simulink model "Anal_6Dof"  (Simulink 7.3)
settings: Solver=ode45  StartTime=0.0  StopTime=500  RelTol=1e-3
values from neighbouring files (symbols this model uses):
  calfa = cos(alfa0*d2r)    [run.m]
  d2r = pi/180    (= 0.0174532925199)    [run.m]
  Kfilt = (wd1^2*wd2^2*wd3^2*wd4^2*wd5^2*wd6^2)/(wn1^2*wn2^2*wn3^2*wn4^2*wn5^2*wn6^2)    (= 0.818930549142)    [run.m]
  klr = lqr(Ap4,Bp4,Q,R)    [run.m]
  kls = lqr(Ap3,Bp3,Q,R)    [run.m]
  salfa = sin(alfa0*d2r)    [run.m]
  Thet0 = 43    [run.m]
  V0 = 18640    [run.m]
  wd1 = 29    [run.m]
  wd2 = 37    [run.m]
  wd3 = 40    [run.m]
  wd4 = 48    [run.m]
  wd5 = 63    [run.m]
  wd6 = 68    [run.m]
  wd7 = 34    [run.m]
  wd8 = 19.1    [run.m]
  wlp = 6.6    [run.m]
  wlp2 = 12    [run.m]
  wlpr = 12    [run.m]
  wn1 = 30    [run.m]
  wn2 = 37.9    [run.m]
  wn3 = 40.2    [run.m]
  wn4 = 48.6    [run.m]
  wn5 = 64    [run.m]
  wn6 = 68.6    [run.m]
  wn7 = 34    [run.m]
  wn8 = 19.1    [run.m]
  zd1 = 0.12    [run.m]
  zd2 = 0.12    [run.m]
  zd3 = 0.1    [run.m]
  zd4 = 0.1    [run.m]
  zd5 = 0.1    [run.m]
  zd6 = 0.1    [run.m]
  zd7 = 0.1    [run.m]
  zd8 = 0.1    [run.m]
  zlp = 0.9    [run.m]
  zlp2 = 0.7    [run.m]
  zlpr = 0.7    [run.m]
  zn1 = 0.008    [run.m]
  zn2 = 0.01    [run.m]
  zn3 = 0.01    [run.m]
  zn4 = 0.02    [run.m]
  zn5 = 0.01    [run.m]
  zn6 = 0.01    [run.m]
  zn7 = 0.01    [run.m]
  zn8 = 0.01    [run.m]
undefined symbols (not defined in the file or in its folder): Aai, Aao, Af, Bai, Bao, Bf, Cai, Cao, Cf, Dai, Dao, Df, KJmix, KSmix

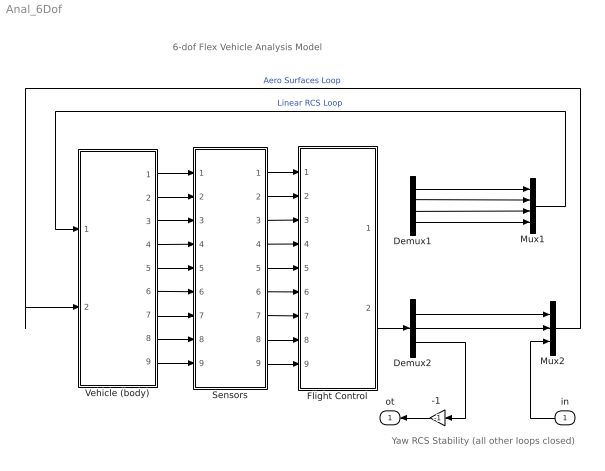
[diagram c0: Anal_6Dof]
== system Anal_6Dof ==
  note: 6-dof Flex Vehicle Analysis Model
  note: Yaw RCS Stability (all other loops closed)
  in : Inport  OutDataType=sfix(16)  OutScaling=2^0
  "-1 " : Gain  Gain=-1  ParameterDataType=sfix(16)  ParameterScaling=2^0  OutDataType=sfix(16)  OutScaling=2^0
  Demux1 : Demux
  Demux2 : Demux  Outputs=3
  Flight Control : Subsystem
  Mux1 : Mux
  Mux2 : Mux  Inputs=3
  Sensors : Subsystem
  Vehicle (body) : Subsystem
  ot : Outport  OutDataType=sfix(16)  OutScaling=2^0
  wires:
  Flight Control/2(Aer_pqr) -> Demux2/1
  Mux2/1 -> Vehicle (body)/2(Aer_pqr)  "Aero Surfaces Loop"
  Mux1/1 -> Vehicle (body)/1(Jet_PQR_Nz)  "Linear RCS Loop"
  Vehicle (body)/1(phi) -> Sensors/1(phi)
  Vehicle (body)/2(p) -> Sensors/2(pb)
  Vehicle (body)/3(r) -> Sensors/3(rb)
  Vehicle (body)/4(bet) -> Sensors/4(beta)
  Vehicle (body)/5(thet) -> Sensors/5(thet)
  Vehicle (body)/6(q) -> Sensors/6(q)
  Vehicle (body)/7(alf) -> Sensors/7(alfa)
  Vehicle (body)/8(Ny) -> Sensors/8(Ny)
  Vehicle (body)/9(Nz) -> Sensors/9(Nz)
  Sensors/1(phio) -> Flight Control/1(phi)
  Sensors/2(pbo) -> Flight Control/2(pb)
  Sensors/3(rbo) -> Flight Control/3(rb)
  Sensors/4(beto) -> Flight Control/4(beta)
  Sensors/5(theto) -> Flight Control/5(thet)
  Sensors/6(qo) -> Flight Control/6(q)
  Sensors/7(alfo) -> Flight Control/7(alfa)
  Sensors/8(Nyo) -> Flight Control/8(Ny)
  Sensors/9(Nzo) -> Flight Control/9(Nz)
  "-1 "/1 -> ot/1
  Demux1/4 -> Mux1/4
  Demux1/1 -> Mux1/1
  Demux2/2 -> Mux2/2
  Demux2/1 -> Mux2/1
  Demux1/2 -> Mux1/2
  Demux2/3 -> "-1 "/1
  in/1 -> Mux2/3
  Demux1/3 -> Mux1/3

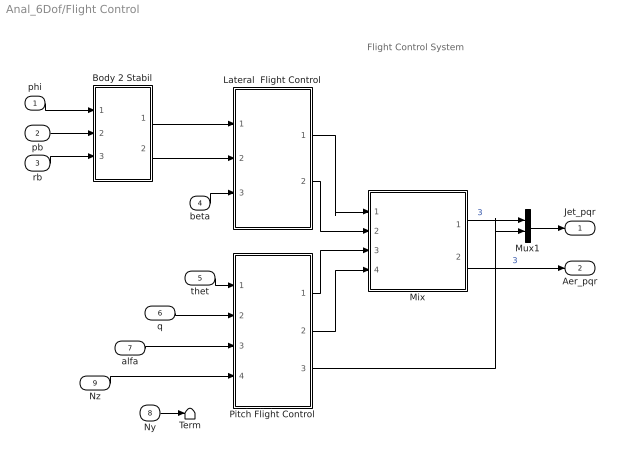
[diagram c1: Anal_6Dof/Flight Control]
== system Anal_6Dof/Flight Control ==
  note: Flight Control System
  phi : Inport  OutDataType=sfix(16)  OutScaling=2^0
  pb : Inport  Port=2  OutDataType=sfix(16)  OutScaling=2^0
  rb : Inport  Port=3  OutDataType=sfix(16)  OutScaling=2^0
  beta : Inport  Port=4  OutDataType=sfix(16)  OutScaling=2^0
  thet : Inport  Port=5  OutDataType=sfix(16)  OutScaling=2^0
  q : Inport  Port=6  OutDataType=sfix(16)  OutScaling=2^0
  alfa : Inport  Port=7  OutDataType=sfix(16)  OutScaling=2^0
  Ny : Inport  Port=8  OutDataType=sfix(16)  OutScaling=2^0
  Nz : Inport  Port=9  OutDataType=sfix(16)  OutScaling=2^0
  Body 2 Stabil : Subsystem
  Lateral  Flight Control : Subsystem
  Mix : Subsystem
  Mux1 : Mux  Inputs=[3,1]
  Pitch Flight Control : Subsystem
  Term : Terminator
  Jet_pqr : Outport  OutDataType=sfix(16)  OutScaling=2^0
  Aer_pqr : Outport  Port=2  OutDataType=sfix(16)  OutScaling=2^0
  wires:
  Lateral  Flight Control/1(rcs_PR) -> Mix/1(Rcs_PR)
  Lateral  Flight Control/2(aero_PR) -> Mix/2(Aer_PR)
  Pitch Flight Control/1(rcs_Q) -> Mix/3(Rcs_Q)
  Pitch Flight Control/2(aero_Q) -> Mix/4(Aer_Q)
  beta/1 -> Lateral  Flight Control/3(beta)
  Mix/2(Aer_pqr) -> Aer_pqr/1  "3"
  thet/1 -> Pitch Flight Control/1(thet)
  q/1 -> Pitch Flight Control/2(q)
  alfa/1 -> Pitch Flight Control/3(alf)
  Body 2 Stabil/2(r_s) -> Lateral  Flight Control/2(rs)
  Body 2 Stabil/1(p_s) -> Lateral  Flight Control/1(ps)
  rb/1 -> Body 2 Stabil/3(r_b)
  pb/1 -> Body 2 Stabil/2(p_b)
  phi/1 -> Body 2 Stabil/1(phi)
  Nz/1 -> Pitch Flight Control/4(Nz)
  Mix/1(Jet_pqr) -> Mux1/1  "3"
  Pitch Flight Control/3(Nzfb) -> Mux1/2
  Mux1/1 -> Jet_pqr/1
  Ny/1 -> Term/1

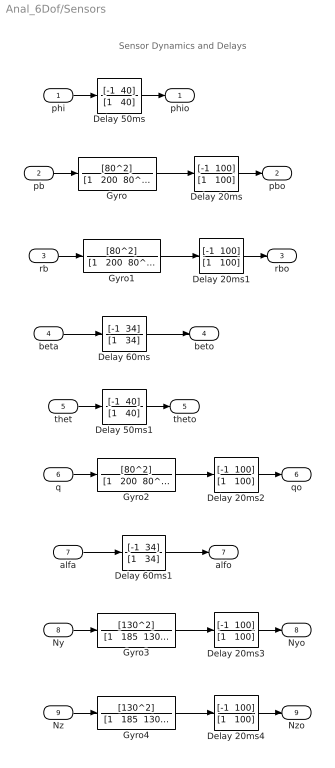
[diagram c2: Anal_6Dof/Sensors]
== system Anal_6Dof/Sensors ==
  note: Sensor Dynamics and Delays
  phi : Inport  OutDataType=sfix(16)  OutScaling=2^0
  pb : Inport  Port=2  OutDataType=sfix(16)  OutScaling=2^0
  rb : Inport  Port=3  OutDataType=sfix(16)  OutScaling=2^0
  beta : Inport  Port=4  OutDataType=sfix(16)  OutScaling=2^0
  thet : Inport  Port=5  OutDataType=sfix(16)  OutScaling=2^0
  q : Inport  Port=6  OutDataType=sfix(16)  OutScaling=2^0
  alfa : Inport  Port=7  OutDataType=sfix(16)  OutScaling=2^0
  Ny : Inport  Port=8  OutDataType=sfix(16)  OutScaling=2^0
  Nz : Inport  Port=9  OutDataType=sfix(16)  OutScaling=2^0
  Delay 20ms{,1..4} (5 alike) : TransferFcn  Numerator="[-1  100]"  Denominator="[1   100]"
  Delay 50ms : TransferFcn  Numerator="[-1  40]"  Denominator="[1   40]"
  Delay 50ms1 : TransferFcn  Numerator="[-1  40]"  Denominator="[1   40]"
  Delay 60ms : TransferFcn  Numerator="[-1  34]"  Denominator="[1   34]"
  Delay 60ms1 : TransferFcn  Numerator="[-1  34]"  Denominator="[1   34]"
  Gyro : TransferFcn  Numerator=[80^2]  Denominator="[1   200  80^2]"
  Gyro1 : TransferFcn  Numerator=[80^2]  Denominator="[1   200  80^2]"
  Gyro2 : TransferFcn  Numerator=[80^2]  Denominator="[1   200  80^2]"
  Gyro3 : TransferFcn  Numerator=[130^2]  Denominator="[1   185  130^2]"
  Gyro4 : TransferFcn  Numerator=[130^2]  Denominator="[1   185  130^2]"
  phio : Outport  OutDataType=sfix(16)  OutScaling=2^0
  pbo : Outport  Port=2  OutDataType=sfix(16)  OutScaling=2^0
  rbo : Outport  Port=3  OutDataType=sfix(16)  OutScaling=2^0
  beto : Outport  Port=4  OutDataType=sfix(16)  OutScaling=2^0
  theto : Outport  Port=5  OutDataType=sfix(16)  OutScaling=2^0
  qo : Outport  Port=6  OutDataType=sfix(16)  OutScaling=2^0
  alfo : Outport  Port=7  OutDataType=sfix(16)  OutScaling=2^0
  Nyo : Outport  Port=8  OutDataType=sfix(16)  OutScaling=2^0
  Nzo : Outport  Port=9  OutDataType=sfix(16)  OutScaling=2^0
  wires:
  Gyro/1 -> Delay 20ms/1
  phi/1 -> Delay 50ms/1
  Delay 50ms/1 -> phio/1
  Delay 20ms/1 -> pbo/1
  pb/1 -> Gyro/1
  Gyro1/1 -> Delay 20ms1/1
  Delay 20ms1/1 -> rbo/1
  rb/1 -> Gyro1/1
  beta/1 -> Delay 60ms/1
  Delay 60ms/1 -> beto/1
  thet/1 -> Delay 50ms1/1
  Delay 50ms1/1 -> theto/1
  Gyro2/1 -> Delay 20ms2/1
  Delay 20ms2/1 -> qo/1
  q/1 -> Gyro2/1
  alfa/1 -> Delay 60ms1/1
  Delay 60ms1/1 -> alfo/1
  Gyro3/1 -> Delay 20ms3/1
  Delay 20ms3/1 -> Nyo/1
  Ny/1 -> Gyro3/1
  Gyro4/1 -> Delay 20ms4/1
  Delay 20ms4/1 -> Nzo/1
  Nz/1 -> Gyro4/1

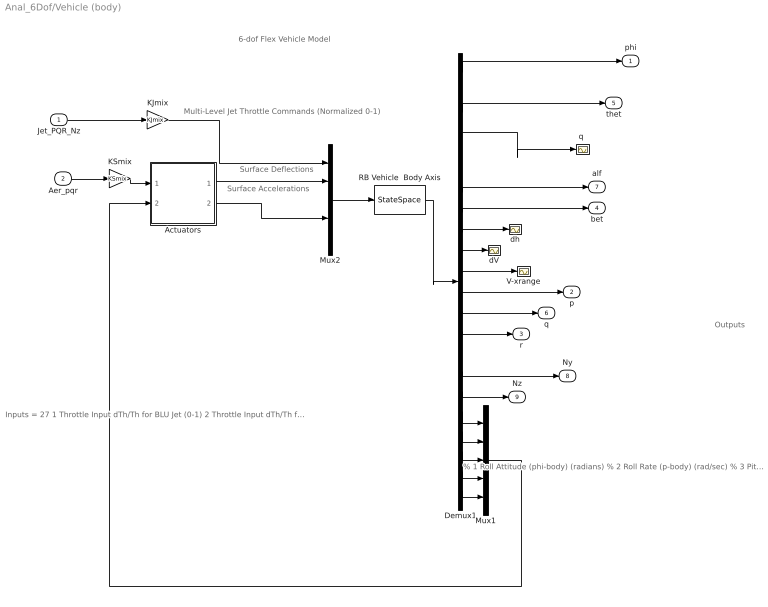
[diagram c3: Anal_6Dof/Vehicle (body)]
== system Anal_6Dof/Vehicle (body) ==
  note: Surface Deflections
  note: Multi-Level Jet Throttle Commands (Normalized 0-1)
  note: % 1 Roll Attitude (phi-body) (radians) % 2 Roll Rate (p-body) (rad/sec) % 3 Pitch Attitude (thet-bdy) (radians) % 4 Pitch Rate (q-body) (rad/sec) % 5 Yaw Attitude (psi-body) (radians) % 6 Yaw Rate (r-body) (rad/sec) % 7 Angle of attack, alfa, (radians) % 8 Angle of sideslip, beta, (radian) % 9 Change in Altitude, delta-h, (feet) % 10 Forward Acceleration (V-dot) (ft/sec) % 11 Cross Range Velocity (Vcr) (ft/sec) % 12 Rate-Gyro # 1, Roll Rate (Body) (rad/sec) % 13 Rate-Gyro # 2, Pitch Rate (Body) (rad/sec) % 14 Rate-Gyro # 3, Yaw Rate (Body) (rad/sec) % 15 Accelerom # 1, (along X), (ft/sec^2) Translat. Acceler % 16 Accelerom # 2, (along Y), (ft/sec^2) Translat. Acceler % 17 Accelerom # 3, (along Z), (ft/sec^2) Translat. Acceler % 18 Hinge Moment for Aero Surface # 1, (ft-lb) % 19 Hinge Moment for Aero Surface # 2, (ft-lb) % 20 Hinge Moment for Aero Surface # 3, (ft-lb) % 21 Hinge Moment for Aero Surface # 4, (ft-lb) % 22 Hinge Moment for Aero Surface # 5, (ft-lb)
  note: 6-dof Flex Vehicle Model
  note: Surface Accelerations
  note: Inputs = 27 1 Throttle Input dTh/Th for BLU Jet (0-1) 2 Throttle Input dTh/Th for BRU Jet (0-1) 3 Throttle Input dTh/Th for BLD Jet (0-1) 4 Throttle Input dTh/Th for BRD Jet (0-1) 5 Throttle Input dTh/Th for BL+Y Jet (0-1) 6 Throttle Input dTh/Th for BR-Y Jet (0-1) 7 Throttle Input dTh/Th for FU Jet (0-1) 8 Throttle Input dTh/Th for FLD Jet (0-1) 9 Throttle Input dTh/Th for FRD Jet (0-1) 10 Throttle Input dTh/Th for FL+Y Jet (0-1) 11 Throttle Input dTh/Th for FR-Y Jet (0-1) 12 Left Outbrd Elevon Deflection (radians) 13 Left Inboard Elevon Deflection (radians) 14 Right Inbrd Elevon Deflection (radians) 15 Right Outbrd Elevon Deflection (radians) 16 Vertical Rudder Deflection (radians) 17 Left Outbrd Elevon Velocity (rad/sec) 18 Left Inboard Elevon Velocity (rad/sec) 19 Right Inbrd Elevon Velocity (rad/sec) 20 Right Outbrd Elevon Velocity (rad/sec) 21 Vertical Rudder Velocity (rad/sec) 22 Left Outbrd Elevon Acceleration (rad/s^2) 23 Left Inboard Elevon Acceleration (rad/s^2) 24 Right Inbrd Elevon Acceleration (rad/s^2) 25 Right Outbrd Elevon Acceleration (rad/s^2) 26 Vertical Rudder Acceleration (rad/s^2) 27 Gust Veloc. Azim,Elev=(45, 90) (deg)
  note: Outputs
  Jet_PQR_Nz : Inport  OutDataType=sfix(16)  OutScaling=2^0
  Aer_pqr : Inport  Port=2  OutDataType=sfix(16)  OutScaling=2^0
  Actuators : Subsystem
  Demux1 : Demux  Outputs=22
  KJmix : Gain  Gain=KJmix  Multiplication=Matrix(K*u)  ParameterDataType=sfix(16)  ParameterScaling=2^0  OutDataType=sfix(16)  OutScaling=2^0
  KSmix : Gain  Gain=KSmix  Multiplication=Matrix(K*u)  ParameterDataType=sfix(16)  ParameterScaling=2^0  OutDataType=sfix(16)  OutScaling=2^0
  Mux1 : Mux  Inputs=5
  Mux2 : Mux  Inputs=[11, 5,5,5, 1]
  RB Vehicle  Body Axis : StateSpace  A=Af  B=Bf  C=Cf  D=Df
  V-xrange : Scope
  dV : Scope
  dh : Scope
  "q " : Scope
  phi : Outport  OutDataType=sfix(16)  OutScaling=2^0
  p : Outport  Port=2  OutDataType=sfix(16)  OutScaling=2^0
  r : Outport  Port=3  OutDataType=sfix(16)  OutScaling=2^0
  bet : Outport  Port=4  OutDataType=sfix(16)  OutScaling=2^0
  thet : Outport  Port=5  OutDataType=sfix(16)  OutScaling=2^0
  q : Outport  Port=6  OutDataType=sfix(16)  OutScaling=2^0
  alf : Outport  Port=7  OutDataType=sfix(16)  OutScaling=2^0
  Ny : Outport  Port=8  OutDataType=sfix(16)  OutScaling=2^0
  Nz : Outport  Port=9  OutDataType=sfix(16)  OutScaling=2^0
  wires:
  Mux2/1 -> RB Vehicle  Body Axis/1
  Demux1/4 -> "q "/1
  Demux1/7 -> alf/1
  Demux1/8 -> bet/1
  Aer_pqr/1 -> KSmix/1
  Demux1/3 -> thet/1
  Demux1/1 -> phi/1
  Demux1/9 -> dh/1
  Demux1/10 -> dV/1
  Demux1/11 -> V-xrange/1
  Jet_PQR_Nz/1 -> KJmix/1
  KJmix/1 -> Mux2/1
  Demux1/12 -> p/1
  Demux1/13 -> q/1
  Demux1/14 -> r/1
  Demux1/17 -> Nz/1
  RB Vehicle  Body Axis/1 -> Demux1/1
  Actuators/1(delta) -> Mux2/2
  KSmix/1 -> Actuators/1(delcom)
  Demux1/16 -> Ny/1
  Actuators/2(delddot) -> Mux2/4
  Demux1/18 -> Mux1/1
  Demux1/19 -> Mux1/2
  Demux1/20 -> Mux1/3
  Demux1/21 -> Mux1/4
  Demux1/22 -> Mux1/5
  Mux1/1 -> Actuators/2(HM)

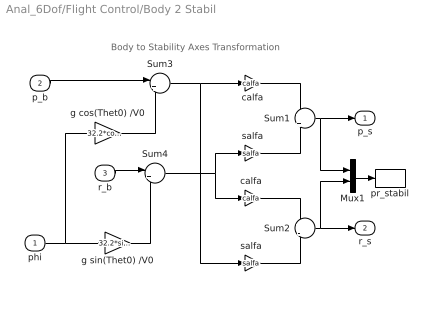
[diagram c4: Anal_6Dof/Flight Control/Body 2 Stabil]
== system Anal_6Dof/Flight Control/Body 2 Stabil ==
  note: Body to Stability Axes Transformation
  phi : Inport  OutDataType=sfix(16)  OutScaling=2^0
  p_b : Inport  Port=2  OutDataType=sfix(16)  OutScaling=2^0
  r_b : Inport  Port=3  OutDataType=sfix(16)  OutScaling=2^0
  Mux1 : Mux  Inputs=2
  Sum1 : Sum  Inputs=+|+  OutDataType=sfix(16)  OutScaling=2^0
  Sum2 : Sum  Inputs=+|-  OutDataType=sfix(16)  OutScaling=2^0
  Sum3 : Sum  Inputs=|++  OutDataType=sfix(16)  OutScaling=2^0
  Sum4 : Sum  Inputs=|+-  OutDataType=sfix(16)  OutScaling=2^0
  calfa : Gain  Gain=calfa  ParameterDataType=sfix(16)  ParameterScaling=2^0  OutDataType=sfix(16)  OutScaling=2^0
  "calfa " : Gain  Gain=calfa  ParameterDataType=sfix(16)  ParameterScaling=2^0  OutDataType=sfix(16)  OutScaling=2^0
  g cos(Thet0) /V0 : Gain  Gain=32.2*cos(Thet0*d2r)/V0  ParameterDataType=sfix(16)  ParameterScaling=2^0  OutDataType=sfix(16)  OutScaling=2^0
  g sin(Thet0) /V0 : Gain  Gain=32.2*sin(Thet0*d2r)/V0  ParameterDataType=sfix(16)  ParameterScaling=2^0  OutDataType=sfix(16)  OutScaling=2^0
  pr_stabil : ToWorkspace  VariableName=pr_st  SampleTime=-1  SaveFormat=Array
  salfa : Gain  Gain=salfa  ParameterDataType=sfix(16)  ParameterScaling=2^0  OutDataType=sfix(16)  OutScaling=2^0
  "salfa " : Gain  Gain=salfa  ParameterDataType=sfix(16)  ParameterScaling=2^0  OutDataType=sfix(16)  OutScaling=2^0
  p_s : Outport  OutDataType=sfix(16)  OutScaling=2^0
  r_s : Outport  Port=2  OutDataType=sfix(16)  OutScaling=2^0
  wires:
  Sum1/1 -> p_s/1, Mux1/1
  Sum2/1 -> r_s/1, Mux1/2
  p_b/1 -> Sum3/1
  r_b/1 -> Sum4/1
  g cos(Thet0) /V0/1 -> Sum3/2
  g sin(Thet0) /V0/1 -> Sum4/2
  phi/1 -> g cos(Thet0) /V0/1, g sin(Thet0) /V0/1
  Sum4/1 -> "calfa "/1, salfa/1
  Sum3/1 -> "salfa "/1, calfa/1
  calfa/1 -> Sum1/1
  salfa/1 -> Sum1/2
  "calfa "/1 -> Sum2/1
  "salfa "/1 -> Sum2/2
  Mux1/1 -> pr_stabil/1

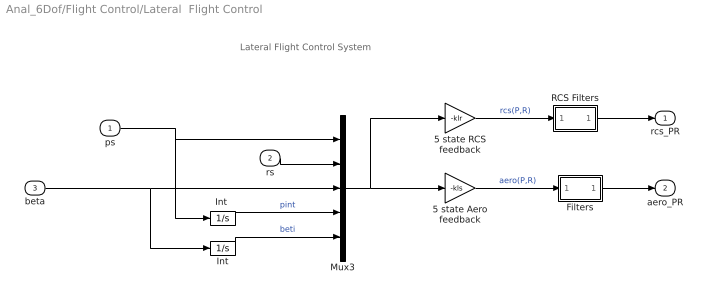
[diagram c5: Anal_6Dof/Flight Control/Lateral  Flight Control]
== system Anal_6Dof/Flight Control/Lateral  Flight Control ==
  note: Lateral Flight Control System
  ps : Inport  OutDataType=sfix(16)  OutScaling=2^0
  rs : Inport  Port=2  OutDataType=sfix(16)  OutScaling=2^0
  beta : Inport  Port=3  OutDataType=sfix(16)  OutScaling=2^0
  5 state Aero feedback : Gain  Gain=-kls  Multiplication=Matrix(K*u)  ParameterDataType=sfix(16)  ParameterScaling=2^0  OutDataType=sfix(16)  OutScaling=2^0
  5 state RCS feedback : Gain  Gain=-klr  Multiplication=Matrix(K*u)  ParameterDataType=sfix(16)  ParameterScaling=2^0  OutDataType=sfix(16)  OutScaling=2^0
  Filters : Subsystem
  Int : Integrator
  "Int " : Integrator
  Mux3 : Mux  Inputs=5
  RCS Filters : Subsystem
  rcs_PR : Outport  OutDataType=sfix(16)  OutScaling=2^0
  aero_PR : Outport  Port=2  OutDataType=sfix(16)  OutScaling=2^0
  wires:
  "Int "/1 -> Mux3/4  "pint"
  Int/1 -> Mux3/5  "beti"
  beta/1 -> Int/1, Mux3/3
  ps/1 -> "Int "/1, Mux3/1
  Mux3/1 -> 5 state Aero feedback/1, 5 state RCS feedback/1
  rs/1 -> Mux3/2
  5 state RCS feedback/1 -> RCS Filters/1(In)  "rcs(P,R)"
  5 state Aero feedback/1 -> Filters/1(In)  "aero(P,R)"
  Filters/1(Ou) -> aero_PR/1
  RCS Filters/1(Ou) -> rcs_PR/1

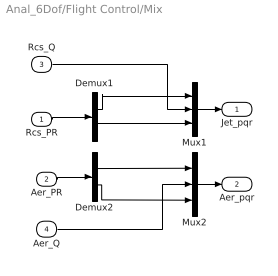
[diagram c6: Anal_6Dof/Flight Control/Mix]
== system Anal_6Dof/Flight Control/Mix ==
  Rcs_PR : Inport  OutDataType=sfix(16)  OutScaling=2^0
  Aer_PR : Inport  Port=2  OutDataType=sfix(16)  OutScaling=2^0
  Rcs_Q : Inport  Port=3  OutDataType=sfix(16)  OutScaling=2^0
  Aer_Q : Inport  Port=4  OutDataType=sfix(16)  OutScaling=2^0
  Demux1 : Demux  Outputs=2
  Demux2 : Demux  Outputs=2
  Mux1 : Mux  Inputs=3
  Mux2 : Mux  Inputs=3
  Jet_pqr : Outport  OutDataType=sfix(16)  OutScaling=2^0
  Aer_pqr : Outport  Port=2  OutDataType=sfix(16)  OutScaling=2^0
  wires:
  Demux1/1 -> Mux1/1
  Demux1/2 -> Mux1/3
  Demux2/1 -> Mux2/1
  Demux2/2 -> Mux2/3
  Mux1/1 -> Jet_pqr/1
  Rcs_PR/1 -> Demux1/1
  Aer_PR/1 -> Demux2/1
  Aer_Q/1 -> Mux2/2
  Mux2/1 -> Aer_pqr/1
  Rcs_Q/1 -> Mux1/2

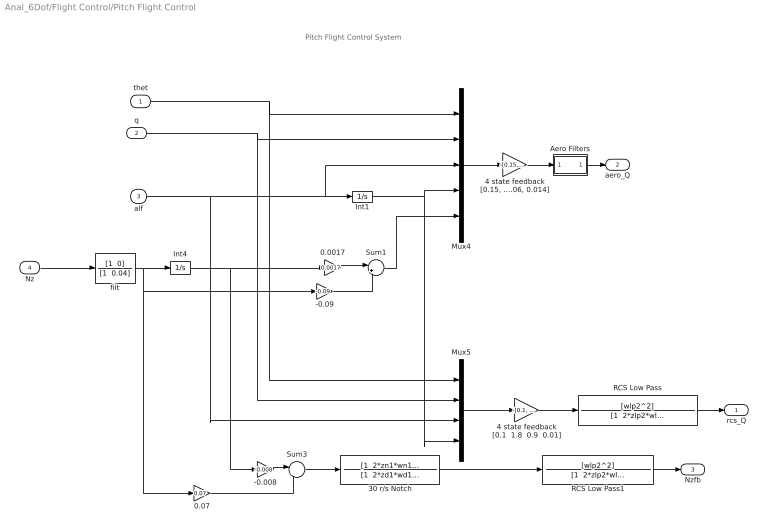
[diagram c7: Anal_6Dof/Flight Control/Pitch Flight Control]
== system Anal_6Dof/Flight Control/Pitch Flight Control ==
  note: Pitch Flight Control System
  thet : Inport  OutDataType=sfix(16)  OutScaling=2^0
  q : Inport  Port=2  OutDataType=sfix(16)  OutScaling=2^0
  alf : Inport  Port=3  OutDataType=sfix(16)  OutScaling=2^0
  Nz : Inport  Port=4  OutDataType=sfix(16)  OutScaling=2^0
  -0.008 : Gain  Gain=-0.008  ParameterDataType=sfix(16)  ParameterScaling=2^0  OutDataType=sfix(16)  OutScaling=2^0
  -0.09 : Gain  Gain=-0.09  ParameterDataType=sfix(16)  ParameterScaling=2^0  OutDataType=sfix(16)  OutScaling=2^0
  0.0017 : Gain  Gain=0.0017  ParameterDataType=sfix(16)  ParameterScaling=2^0  OutDataType=sfix(16)  OutScaling=2^0
  0.07 : Gain  Gain=0.07  ParameterDataType=sfix(16)  ParameterScaling=2^0  OutDataType=sfix(16)  OutScaling=2^0
  30 r/s Notch : TransferFcn  Numerator="[1  2*zn1*wn1  wn1^2]"  Denominator="[1  2*zd1*wd1  wd1^2]"
  4 state feedback [0.1  1.8  0.9  0.01] : Gain  Gain="-[0.1,   1.8,   0.9,    0.01]"  Multiplication=Matrix(K*u)  ParameterDataType=sfix(16)  ParameterScaling=2^0  OutDataType=sfix(16)  OutScaling=2^0
  "4 state feedback [0.15, 2, 0.9, 0.06, 0.014]" : Gain  Gain="-[0.15,   2,   0.9,    0.06,   0.015]"  Multiplication=Matrix(K*u)  ParameterDataType=sfix(16)  ParameterScaling=2^0  OutDataType=sfix(16)  OutScaling=2^0
  Aero Filters : Subsystem
  Int1 : Integrator
  Int4 : Integrator
  Mux4 : Mux  Inputs=5
  Mux5 : Mux
  RCS Low Pass : TransferFcn  Numerator=[wlp2^2]  Denominator="[1  2*zlp2*wlp2  wlp2^2]"
  RCS Low Pass1 : TransferFcn  Numerator=[wlp2^2]  Denominator="[1  2*zlp2*wlp2  wlp2^2]"
  Sum1 : Sum  Inputs=|++  OutDataType=sfix(16)  OutScaling=2^0
  Sum3 : Sum  Inputs=|++  OutDataType=sfix(16)  OutScaling=2^0
  filt : TransferFcn  Numerator="[1  0]"  Denominator="[1  0.04]"
  rcs_Q : Outport  OutDataType=sfix(16)  OutScaling=2^0
  aero_Q : Outport  Port=2  OutDataType=sfix(16)  OutScaling=2^0
  Nzfb : Outport  Port=3  OutDataType=sfix(16)  OutScaling=2^0
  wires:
  alf/1 -> Mux5/3, Mux4/3, Int1/1
  filt/1 -> 0.07/1, -0.09/1, Int4/1
  Int4/1 -> -0.008/1, 0.0017/1
  -0.008/1 -> Sum3/1
  0.07/1 -> Sum3/2
  4 state feedback [0.1  1.8  0.9  0.01]/1 -> RCS Low Pass/1
  Mux5/1 -> 4 state feedback [0.1  1.8  0.9  0.01]/1
  "4 state feedback [0.15, 2, 0.9, 0.06, 0.014]"/1 -> Aero Filters/1(in)
  Mux4/1 -> "4 state feedback [0.15, 2, 0.9, 0.06, 0.014]"/1
  Sum1/1 -> Mux4/5
  Nz/1 -> filt/1
  -0.09/1 -> Sum1/2
  0.0017/1 -> Sum1/1
  q/1 -> Mux5/2, Mux4/2
  thet/1 -> Mux5/1, Mux4/1
  Int1/1 -> Mux5/4, Mux4/4
  Sum3/1 -> 30 r/s Notch/1
  Aero Filters/1(ot) -> aero_Q/1
  RCS Low Pass/1 -> rcs_Q/1
  RCS Low Pass1/1 -> Nzfb/1
  30 r/s Notch/1 -> RCS Low Pass1/1

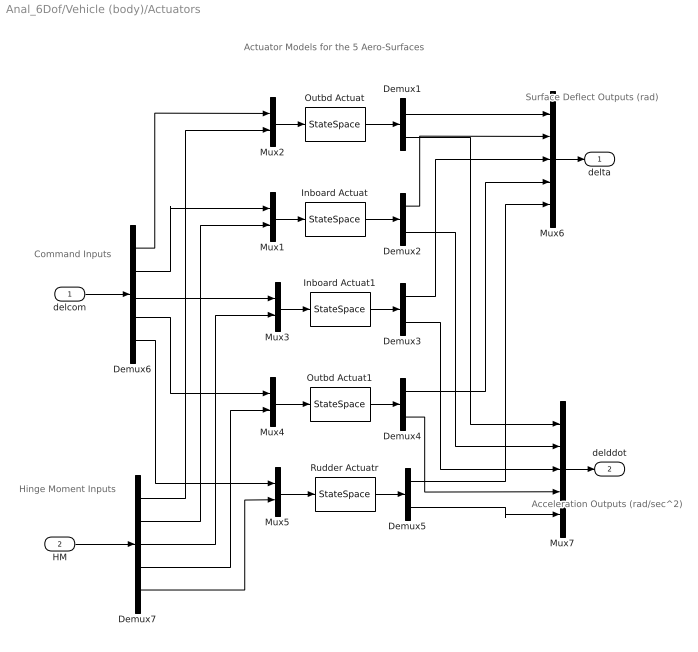
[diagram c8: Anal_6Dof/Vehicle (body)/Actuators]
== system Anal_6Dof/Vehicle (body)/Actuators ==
  note: Command Inputs
  note: Hinge Moment Inputs
  note: Actuator Models for the 5 Aero-Surfaces
  note: Acceleration Outputs (rad/sec^2)
  note: Surface Deflect Outputs (rad)
  delcom : Inport  OutDataType=sfix(16)  OutScaling=2^0
  HM : Inport  Port=2  OutDataType=sfix(16)  OutScaling=2^0
  Demux{1..5} (5 alike) : Demux  Outputs=3
  Demux6 : Demux  Outputs=5
  Demux7 : Demux  Outputs=5
  Inboard Actuat : StateSpace  A=Aai  B=Bai  C=Cai  D=Dai
  Inboard Actuat1 : StateSpace  A=Aai  B=Bai  C=Cai  D=Dai
  Mux{1..5} (5 alike) : Mux  Inputs=2
  Mux6 : Mux  Inputs=5
  Mux7 : Mux  Inputs=5
  Outbd Actuat : StateSpace  A=Aao  B=Bao  C=Cao  D=Dao
  Outbd Actuat1 : StateSpace  A=Aao  B=Bao  C=Cao  D=Dao
  Rudder Actuatr : StateSpace  A=Aai  B=Bai  C=Cai  D=Dai
  delta : Outport  OutDataType=sfix(16)  OutScaling=2^0
  delddot : Outport  Port=2  OutDataType=sfix(16)  OutScaling=2^0
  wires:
  Mux6/1 -> delta/1
  Mux7/1 -> delddot/1
  Mux1/1 -> Inboard Actuat/1
  Mux2/1 -> Outbd Actuat/1
  Mux3/1 -> Inboard Actuat1/1
  Mux4/1 -> Outbd Actuat1/1
  Mux5/1 -> Rudder Actuatr/1
  Outbd Actuat/1 -> Demux1/1
  Inboard Actuat/1 -> Demux2/1
  Inboard Actuat1/1 -> Demux3/1
  Outbd Actuat1/1 -> Demux4/1
  Rudder Actuatr/1 -> Demux5/1
  delcom/1 -> Demux6/1
  Demux6/1 -> Mux2/1
  Demux6/2 -> Mux1/1
  Demux6/3 -> Mux3/1
  Demux6/4 -> Mux4/1
  Demux6/5 -> Mux5/1
  Demux5/3 -> Mux7/5
  Demux4/3 -> Mux7/4
  Demux3/3 -> Mux7/3
  Demux2/3 -> Mux7/2
  Demux1/3 -> Mux7/1
  Demux1/1 -> Mux6/1
  Demux2/1 -> Mux6/2
  Demux3/1 -> Mux6/3
  Demux4/1 -> Mux6/4
  Demux5/1 -> Mux6/5
  Demux7/1 -> Mux2/2
  Demux7/2 -> Mux1/2
  Demux7/3 -> Mux3/2
  Demux7/4 -> Mux4/2
  Demux7/5 -> Mux5/2
  HM/1 -> Demux7/1

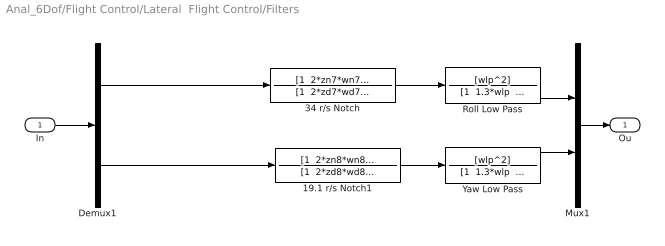
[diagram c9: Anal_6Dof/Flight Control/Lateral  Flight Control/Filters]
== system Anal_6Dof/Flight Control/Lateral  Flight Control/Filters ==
  In : Inport  OutDataType=sfix(16)  OutScaling=2^0
  19.1 r/s Notch1 : TransferFcn  Numerator="[1  2*zn8*wn8  wn8^2]"  Denominator="[1  2*zd8*wd8  wd8^2]"
  34 r/s Notch : TransferFcn  Numerator="[1  2*zn7*wn7  wn7^2]"  Denominator="[1  2*zd7*wd7  wd7^2]"
  Demux1 : Demux  Outputs=2
  Mux1 : Mux  Inputs=2
  Roll Low Pass : TransferFcn  Numerator=[wlp^2]  Denominator="[1  1.3*wlp  wlp^2]"
  Yaw Low Pass : TransferFcn  Numerator=[wlp^2]  Denominator="[1  1.3*wlp  wlp^2]"
  Ou : Outport  OutDataType=sfix(16)  OutScaling=2^0
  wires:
  In/1 -> Demux1/1
  Demux1/1 -> 34 r/s Notch/1
  Mux1/1 -> Ou/1
  Roll Low Pass/1 -> Mux1/1
  Demux1/2 -> 19.1 r/s Notch1/1
  Yaw Low Pass/1 -> Mux1/2
  34 r/s Notch/1 -> Roll Low Pass/1
  19.1 r/s Notch1/1 -> Yaw Low Pass/1

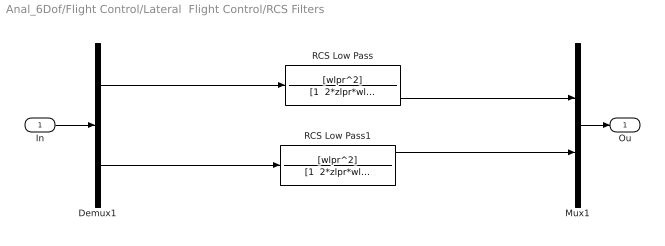
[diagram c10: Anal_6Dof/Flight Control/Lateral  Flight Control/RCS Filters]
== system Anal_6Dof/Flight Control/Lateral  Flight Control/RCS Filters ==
  In : Inport  OutDataType=sfix(16)  OutScaling=2^0
  Demux1 : Demux  Outputs=2
  Mux1 : Mux  Inputs=2
  RCS Low Pass : TransferFcn  Numerator=[wlpr^2]  Denominator="[1  2*zlpr*wlpr  wlpr^2]"
  RCS Low Pass1 : TransferFcn  Numerator=[wlpr^2]  Denominator="[1  2*zlpr*wlpr  wlpr^2]"
  Ou : Outport  OutDataType=sfix(16)  OutScaling=2^0
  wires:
  In/1 -> Demux1/1
  Demux1/1 -> RCS Low Pass/1
  Mux1/1 -> Ou/1
  Demux1/2 -> RCS Low Pass1/1
  RCS Low Pass/1 -> Mux1/1
  RCS Low Pass1/1 -> Mux1/2

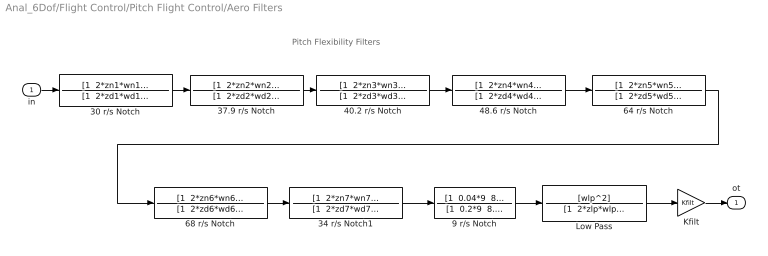
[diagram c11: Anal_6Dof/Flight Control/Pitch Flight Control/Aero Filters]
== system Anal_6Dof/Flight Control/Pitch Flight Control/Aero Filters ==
  note: Pitch Flexibility Filters
  in : Inport  OutDataType=sfix(16)  OutScaling=2^0
  30 r/s Notch : TransferFcn  Numerator="[1  2*zn1*wn1  wn1^2]"  Denominator="[1  2*zd1*wd1  wd1^2]"
  34 r/s Notch1 : TransferFcn  Numerator="[1  2*zn7*wn7  wn7^2]"  Denominator="[1  2*zd7*wd7  wd7^2]"
  37.9 r/s Notch : TransferFcn  Numerator="[1  2*zn2*wn2  wn2^2]"  Denominator="[1  2*zd2*wd2  wd2^2]"
  40.2 r/s Notch : TransferFcn  Numerator="[1  2*zn3*wn3  wn3^2]"  Denominator="[1  2*zd3*wd3  wd3^2]"
  48.6 r/s Notch : TransferFcn  Numerator="[1  2*zn4*wn4  wn4^2]"  Denominator="[1  2*zd4*wd4  wd4^2]"
  64 r/s Notch : TransferFcn  Numerator="[1  2*zn5*wn5  wn5^2]"  Denominator="[1  2*zd5*wd5  wd5^2]"
  68 r/s Notch : TransferFcn  Numerator="[1  2*zn6*wn6  wn6^2]"  Denominator="[1  2*zd6*wd6  wd6^2]"
  9 r/s Notch : TransferFcn  Numerator="[1  0.04*9  8.5^2]"  Denominator="[1  0.2*9  8.5^2]"
  Kfilt : Gain  Gain=Kfilt  ParameterDataType=sfix(16)  ParameterScaling=2^0  OutDataType=sfix(16)  OutScaling=2^0
  Low Pass : TransferFcn  Numerator=[wlp^2]  Denominator="[1  2*zlp*wlp  wlp^2]"
  ot : Outport  OutDataType=sfix(16)  OutScaling=2^0
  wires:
  in/1 -> 30 r/s Notch/1
  30 r/s Notch/1 -> 37.9 r/s Notch/1
  37.9 r/s Notch/1 -> 40.2 r/s Notch/1
  40.2 r/s Notch/1 -> 48.6 r/s Notch/1
  Kfilt/1 -> ot/1
  68 r/s Notch/1 -> 34 r/s Notch1/1
  Low Pass/1 -> Kfilt/1
  48.6 r/s Notch/1 -> 64 r/s Notch/1
  64 r/s Notch/1 -> 68 r/s Notch/1
  9 r/s Notch/1 -> Low Pass/1
  34 r/s Notch1/1 -> 9 r/s Notch/1
